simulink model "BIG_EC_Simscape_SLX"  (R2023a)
settings: Solver=ode23s  StartTime=0.0  StopTime=10.0  MaxStep=0.001  RelTol=1e-3
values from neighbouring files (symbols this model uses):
  C_3 = 0.001*F    (= 0.001)    [BIG_EC_Simscape_EQN.m]    (also in BIG_EC_Simscape_SLX_m.m; Electric_Circuit_03_EQN.m; Electric_Circuit_03_SLX_m.m; Electric_Circuit_07_EQN.m)
  C_8 = 0.001*F    (= 0.001)    [BIG_EC_Simscape_EQN.m]    (also in BIG_EC_Simscape_SLX_m.m; Electric_Circuit_11_EQN.m; Electric_Circuit_11_SLX_m.m; Hydraulic_Circuit_03_EQN.m)
  C_c = 0.001*F    (= 0.001)    [BIG_EC_Simscape_EQN.m]    (also in BIG_EC_Simscape_SLX_m.m)
  C_d = 0.001*F    (= 0.001)    [BIG_EC_Simscape_EQN.m]    (also in BIG_EC_Simscape_SLX_m.m)
  I_5_0 = 0*A    (= 0)    [BIG_EC_Simscape_SLX_m.m]    (also in Electric_Circuit_01_SLX_m.m; Electric_Circuit_06_SLX_m.m; Electric_Circuit_09_SLX_m.m; Electric_Circuit_10_SLX_m.m)
  I_9_0 = 0*A    (= 0)    [BIG_EC_Simscape_SLX_m.m]    (also in Electric_Circuit_10_SLX_m.m; Electric_Circuit_11_SLX_m.m)
  I_e_0 = 0*A    (= 0)    [BIG_EC_Simscape_SLX_m.m]
  I_g_0 = 0*A    (= 0)    [BIG_EC_Simscape_SLX_m.m]
  L_5 = 0.002*H    (= 0.002)    [BIG_EC_Simscape_EQN.m]    (also in BIG_EC_Simscape_SLX_m.m; Electric_Circuit_01_EQN.m; Electric_Circuit_01_SLX_m.m; Electric_Circuit_06_EQN.m)
  L_9 = 0.002*H    (= 0.002)    [BIG_EC_Simscape_EQN.m]    (also in BIG_EC_Simscape_SLX_m.m; Electric_Circuit_11_EQN.m; Electric_Circuit_11_SLX_m.m)
  L_g = 0.002*H    (= 0.002)    [BIG_EC_Simscape_EQN.m]    (also in BIG_EC_Simscape_SLX_m.m)
  R_2 = 100*Ohm    (= 100)    [BIG_EC_Simscape_EQN.m]    (also in BIG_EC_Simscape_SLX_m.m; Electric_Circuit_07_EQN.m; Electric_Circuit_07_SLX_m.m; Electric_Circuit_10_EQN.m)
  R_4 = 100*Ohm    (= 100)    [BIG_EC_Simscape_EQN.m]    (also in BIG_EC_Simscape_SLX_m.m; Electric_Circuit_08_EQN.m; Electric_Circuit_08_SLX_m.m; Electric_Circuit_10_EQN.m)
  R_6 = 100*Ohm    (= 100)    [BIG_EC_Simscape_EQN.m]    (also in BIG_EC_Simscape_SLX_m.m; Electric_Circuit_02_EQN.m; Electric_Circuit_02_SLX_m.m; Electric_Circuit_04_EQN.m)
  R_7 = 100*Ohm    (= 100)    [BIG_EC_Simscape_EQN.m]    (also in BIG_EC_Simscape_SLX_m.m; Electric_Circuit_03_EQN.m; Electric_Circuit_03_SLX_m.m; Electric_Circuit_06_EQN.m)
  R_f = 100*Ohm    (= 100)    [BIG_EC_Simscape_EQN.m]    (also in BIG_EC_Simscape_SLX_m.m; Electrical_DC_Motor_Pump_and_Load_EQN.m = 10000; Electrical_DC_Motor_Pump_and_Load_SLX_m.m = 10000)
  R_h = 100*Ohm    (= 100)    [BIG_EC_Simscape_EQN.m]    (also in BIG_EC_Simscape_SLX_m.m)
  R_i = 100*Ohm    (= 100)    [BIG_EC_Simscape_EQN.m]    (also in BIG_EC_Simscape_SLX_m.m)
  Ts = Tfin/Nr_Ts_Points    (= 0.0003)    [BIG_EC_Simscape_SLX_m.m]    (also in Car_Dumper_SLX_m.m = 0.0022779; Electric_Circuit_01_SLX_m.m = 0.005; Electric_Circuit_02_SLX_m.m = 0.000480145; Electric_Circuit_03_SLX_m.m = 0.0006)
  V_1_0 = 10*V    (= 10)    [BIG_EC_Simscape_SLX_m.m]    (also in Electric_Circuit_02_SLX_m.m; Electric_Circuit_03_SLX_m.m; Electric_Circuit_04_SLX_m.m; Electric_Circuit_05_SLX_m.m)
  V_3_0 = 0*V    (= 0)    [BIG_EC_Simscape_SLX_m.m]    (also in Electric_Circuit_03_SLX_m.m; Electric_Circuit_07_SLX_m.m; Electric_Circuit_11_SLX_m.m; Electrical_Transformer_SLX_m.m)
  V_8_0 = 0*V    (= 0)    [BIG_EC_Simscape_SLX_m.m]    (also in Electric_Circuit_03_SLX_m.m; Electric_Circuit_04_SLX_m.m; Electric_Circuit_09_SLX_m.m; Electric_Circuit_11_SLX_m.m)
  V_b_0 = 0*V    (= 0)    [BIG_EC_Simscape_SLX_m.m]
  V_c_0 = 0*V    (= 0)    [BIG_EC_Simscape_SLX_m.m]
  V_d_0 = 0*V    (= 0)    [BIG_EC_Simscape_SLX_m.m]

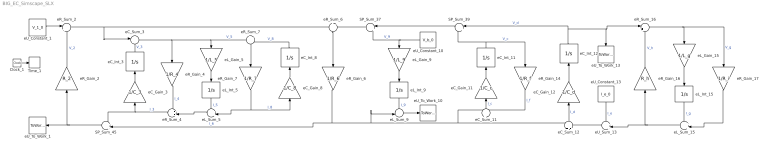
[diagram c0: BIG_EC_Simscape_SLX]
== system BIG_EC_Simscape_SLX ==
  Clock_1 : Clock
  SP_Sum_37 : Sum  Inputs=|++
  SP_Sum_39 : Sum  Inputs=|++
  SP_Sum_45 : Sum  Inputs=++|
  Time_1 : ToWorkspace  VariableName=t  SaveFormat=Timeseries  SampleTime=Ts
  eC_Gain_11 : Gain  Gain=1/C_c  Multiplication=Matrix(K*u)
  eC_Gain_12 : Gain  Gain=1/C_d  Multiplication=Matrix(K*u)
  eC_Gain_3 : Gain  Gain=1/C_3  Multiplication=Matrix(K*u)
  eC_Gain_8 : Gain  Gain=1/C_8  Multiplication=Matrix(K*u)
  eC_Int_11 : Integrator  InitialCondition=V_c_0
  eC_Int_12 : Integrator  InitialCondition=V_d_0
  eC_Int_3 : Integrator  InitialCondition=V_3_0
  eC_Int_8 : Integrator  InitialCondition=V_8_0
  eC_Sum_11 : Sum  Inputs=+|-
  eC_Sum_12 : Sum  Inputs=+|-
  eC_Sum_3 : Sum  Inputs=|+-
  eL_Gain_15 : Gain  Gain=1/L_g  Multiplication=Matrix(K*u)
  eL_Gain_5 : Gain  Gain=1/L_5  Multiplication=Matrix(K*u)
  eL_Gain_9 : Gain  Gain=1/L_9  Multiplication=Matrix(K*u)
  eL_Int_15 : Integrator  InitialCondition=I_g_0
  eL_Int_5 : Integrator  InitialCondition=I_5_0
  eL_Int_9 : Integrator  InitialCondition=I_9_0
  eL_Sum_15 : Sum  Inputs=++|
  eL_Sum_5 : Sum  Inputs=++|
  eL_Sum_9 : Sum  Inputs=-+|
  eR_Gain_14 : Gain  Gain=1/R_f  Multiplication=Matrix(K*u)
  eR_Gain_16 : Gain  Gain=R_h  Multiplication=Matrix(K*u)
  eR_Gain_17 : Gain  Gain=1/R_i  Multiplication=Matrix(K*u)
  eR_Gain_2 : Gain  Gain=R_2  Multiplication=Matrix(K*u)
  eR_Gain_4 : Gain  Gain=1/R_4  Multiplication=Matrix(K*u)
  eR_Gain_6 : Gain  Gain=1/R_6  Multiplication=Matrix(K*u)
  eR_Gain_7 : Gain  Gain=1/R_7  Multiplication=Matrix(K*u)
  eR_Sum_16 : Sum  Inputs=|+-
  eR_Sum_2 : Sum  Inputs=|+-
  eR_Sum_4 : Sum  Inputs=++|
  eR_Sum_6 : Sum  Inputs=+|-
  eR_Sum_7 : Sum  Inputs=+|-
  eU_Constant_1 : Constant  Value=V_1_0
  eU_Constant_10 : Constant  Value=V_b_0
  eU_Constant_13 : Constant  Value=I_e_0
  eU_Sum_13 : Sum  Inputs=++|
  eU_To_Work_1 : ToWorkspace  VariableName=I_1_0  SaveFormat=Timeseries  SampleTime=Ts
  eU_To_Work_10 : ToWorkspace  VariableName=I_b_0  SaveFormat=Timeseries  SampleTime=Ts
  eU_To_Work_13 : ToWorkspace  VariableName=V_e_0  SaveFormat=Timeseries  SampleTime=Ts
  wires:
  eU_Constant_1/1 -> eR_Sum_2/1
  eR_Sum_2/1 -> eC_Sum_3/1, eR_Sum_6/1
  SP_Sum_45/1 -> eU_To_Work_1/1, eR_Gain_2/1
  eR_Gain_2/1 -> eR_Sum_2/2  "V_2"
  eR_Gain_6/1 -> SP_Sum_45/2, eL_Sum_9/2, eC_Sum_11/1, eC_Sum_12/1  "I_6"
  eR_Sum_4/1 -> SP_Sum_45/1, eC_Gain_3/1  "I_3"
  eC_Sum_3/1 -> eR_Gain_4/1, eL_Gain_5/1, eR_Sum_7/1  "V_5"
  eC_Gain_3/1 -> eC_Int_3/1
  eC_Int_3/1 -> eC_Sum_3/2  "V_3"
  eL_Sum_5/1 -> eR_Sum_4/2
  eR_Gain_4/1 -> eR_Sum_4/1  "I_4"
  eR_Gain_7/1 -> eL_Sum_5/2, eC_Gain_8/1  "I_8"
  eL_Gain_5/1 -> eL_Int_5/1
  eL_Int_5/1 -> eL_Sum_5/1  "I_5"
  eC_Int_8/1 -> eR_Sum_7/2  "V_8"
  eR_Sum_7/1 -> eR_Gain_7/1
  eC_Gain_8/1 -> eC_Int_8/1
  SP_Sum_37/1 -> eR_Sum_6/2
  eR_Sum_6/1 -> eR_Gain_6/1
  SP_Sum_39/1 -> SP_Sum_37/1
  eU_Constant_10/1 -> SP_Sum_37/2, eL_Gain_9/1  "V_9"
  eL_Sum_9/1 -> eU_To_Work_10/1
  eL_Gain_9/1 -> eL_Int_9/1
  eL_Int_9/1 -> eL_Sum_9/1  "I_9"
  eC_Int_12/1 -> SP_Sum_39/1, eU_To_Work_13/1, eR_Sum_16/1  "V_d"
  eC_Int_11/1 -> SP_Sum_39/2, eR_Gain_14/1  "V_c"
  eR_Gain_14/1 -> eC_Sum_11/2  "I_f"
  eC_Sum_11/1 -> eC_Gain_11/1  "I_c"
  eC_Gain_11/1 -> eC_Int_11/1
  eU_Sum_13/1 -> eC_Sum_12/2
  eC_Sum_12/1 -> eC_Gain_12/1  "I_d"
  eC_Gain_12/1 -> eC_Int_12/1
  eL_Sum_15/1 -> eU_Sum_13/2, eR_Gain_16/1
  eU_Constant_13/1 -> eU_Sum_13/1  "I_e"
  eR_Sum_16/1 -> eL_Gain_15/1, eR_Gain_17/1  "V_g"
  eR_Gain_16/1 -> eR_Sum_16/2  "V_h"
  eR_Gain_17/1 -> eL_Sum_15/2  "I_i"
  eL_Gain_15/1 -> eL_Int_15/1
  eL_Int_15/1 -> eL_Sum_15/1  "I_g"
  Clock_1/1 -> Time_1/1
